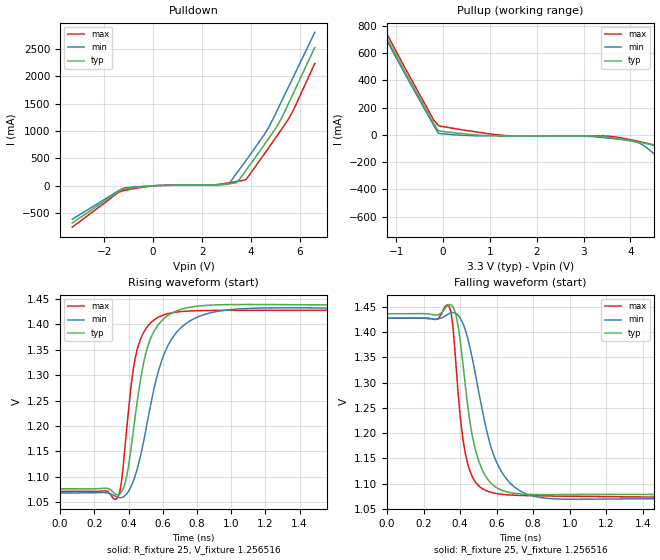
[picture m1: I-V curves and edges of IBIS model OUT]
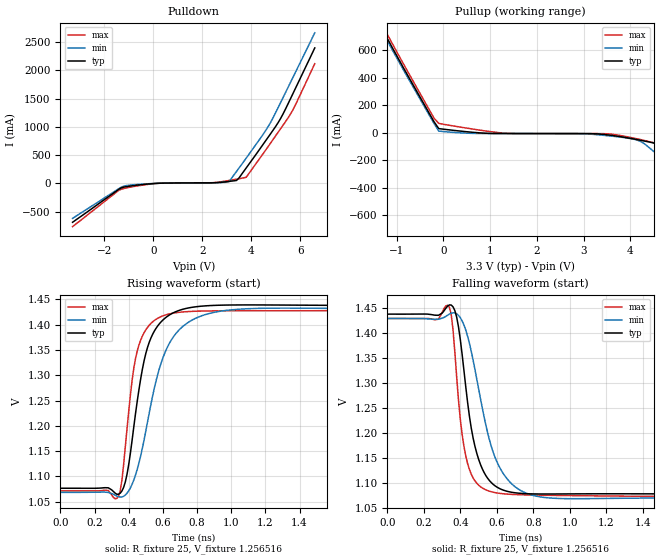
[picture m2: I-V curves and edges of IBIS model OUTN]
|   IBIS File of SG2520VHN C
|   LVDS, Vcc=3.3V, Io=7mA, fo>212.5MHz
[IBIS Ver]   3.2
[File Name]   sg2520vhn_hf_7m_33v.ibs
[File Rev]   1.0
[Date]   July 30, 2020
[Source]
Fairchild Ensigna Lab's Method
[Notes]
Created by Minoru Kozaki
[Disclaimer]
Seiko Epson Corporation makes no warranty with respect to the
information contained herein.
[Copyright]
Copyright(C) 2020, Seiko Epson Corporation. All rights reserved.
|   Component
[Component]   SG2520VHN
[Manufacturer]  Seiko Epson Corporation
[Package]
R_pkg   17.7m   NA   NA
L_pkg   235p   NA   NA
C_pkg   208f   NA   NA
[Pin]   signal_name   model_name   R_pin   L_pin   C_pin
1   OE/ST   NC
2   NC   NC
3   GND   GND
4   OUT   OUT   17.7m   235p   208f
5   OUTN   OUTN   10.4m   129p   221f
6   VCC   POWER
[Diff Pin] inv_pin  vdiff  tdelay_typ
4   5   0   0
| Models and submodels in the file (2): OUT (Output), OUTN (Output)
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|   Model OUT
[Model]   OUT
Model_type   Output
Polarity   Non-Inverting
Vref = 1.25
Vmeas = 1.25
Rref = 25
Cref = 0
C_comp   4.5p   4.5p   4.5p
[Temperature Range]   25   105   -40
[Voltage Range]   3.3   2.97   3.63
[Pullup Reference]   3.3   2.97   3.63
[Pulldown Reference]   0   0   0
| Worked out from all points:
|   slope of the pulldown table from 0 to 0.495 V, typ, clamps not added: 60.1 ohm
|   slope of the pullup table from 0 to 0.495 V, typ, clamps not added: 26.8 ohm
|   falling waveform, R_fixture 25, V_fixture 1.256516: 20-80 % time 92ps typ, 140ps min, 66ps max; typ from 1.44 V to 1.08 V
|   rising waveform, R_fixture 25, V_fixture 1.256516: 20-80 % time 109ps typ, 158ps min, 81.2ps max; typ from 1.08 V to 1.44 V
[Pullup]
-3.3V     2.52A      2.492A     2.553A
-1.4V     837.1mA    817.7mA    870.6mA
-1.3V     772.7mA    753.7mA    805.3mA
-1.2V     708.4mA    690.2mA    740mA
-200mV    81.14mA    68.43mA    107.5mA
-100mV    28.99mA    10.87mA    66.98mA
1.3V      -6.928mA   -7.066mA   -4.25mA
3.7V      -25.31mA   -29.45mA   -16.55mA
4.2V      -55.06mA   -61.12mA   -49.68mA
4.6V      -88.94mA   -164.9mA   -82.59mA
5.1V      -237.8mA   -305.4mA   -156.3mA
6.6V      -698.2mA   -717.4mA   -668.6mA
[Pulldown]
-3.3V     -683.2mA   -614.5mA   -759.8mA
-1.3V     -78.51mA   -64.83mA   -102.6mA
-900mV    -45.62mA   -28.83mA   -63.64mA
100mV     -996uA     -459.2uA   -2.878mA
2.4V      9.207mA    8.749mA    11.16mA
3.1V      34.38mA    33.73mA    50.95mA
3.4V      51.2mA     217.7mA    74.09mA
3.8V      283.8mA    464.4mA    112mA
4.6V      786.4mA    975.9mA    614.4mA
5.2V      1.197A     1.498A     999.8mA
5.7V      1.663A     1.963A     1.357A
6.6V      2.523A     2.802A     2.232A
[Falling Waveform]
R_fixture = 25
V_fixture = 1.256516
V_fixture_min = 1.247959
V_fixture_max = 1.249678
0s        1.437V     1.428V     1.428V
340ps     1.455V     1.437V     1.452V
380ps     1.43V      1.437V     1.323V
410ps     1.355V     1.422V     1.203V
440ps     1.259V     1.39V      1.141V
500ps     1.147V     1.286V     1.096V
580ps     1.097V     1.16V      1.082V
700ps     1.08V      1.092V     1.077V
900ps     1.078V     1.07V      1.075V
4ns       1.077V     1.069V     1.072V
[Rising Waveform]
R_fixture = 25
V_fixture = 1.256516
V_fixture_min = 1.247959
V_fixture_max = 1.249678
0s        1.076V     1.068V     1.071V
320ps     1.067V     1.062V     1.056V
360ps     1.07V      1.059V     1.094V
420ps     1.169V     1.085V     1.293V
450ps     1.246V     1.115V     1.35V
520ps     1.364V     1.226V     1.4V
630ps     1.417V     1.358V     1.421V
780ps     1.435V     1.411V     1.427V
1.05ns    1.439V     1.43V      1.428V
4ns       1.437V     1.428V     1.428V
[Ramp]
R_load = 25
dV/dt_r   0.21562/108.00p   0.21479/156.49p   0.21376/80.76p
dV/dt_f   0.21562/91.62p   0.21479/139.10p   0.21376/65.76p
|   Model OUTN
[Model]   OUTN
Model_type   Output
Polarity   Inverting
Vref = 1.250
Vmeas = 1.250
Rref = 25
Cref = 0
C_comp   4.5p   4.5p   4.5p
[Temperature Range]   25   105   -40
[Voltage Range]   3.3   2.97   3.63
[Pullup Reference]   3.3   2.97   3.63
[Pulldown Reference]   0   0   0
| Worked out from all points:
|   slope of the pulldown table from 0 to 0.495 V, typ, clamps not added: 60 ohm
|   slope of the pullup table from 0 to 0.495 V, typ, clamps not added: 26.9 ohm
|   falling waveform, R_fixture 25, V_fixture 1.256516: 20-80 % time 91.9ps typ, 139ps min, 66.3ps max; typ from 1.44 V to 1.08 V
|   rising waveform, R_fixture 25, V_fixture 1.256516: 20-80 % time 109ps typ, 158ps min, 81.5ps max; typ from 1.08 V to 1.44 V
[Pullup]
-3.3V     2.395A     2.372A     2.423A
-1.4V     808.1mA    789.2mA    840.5mA
-1.3V     745.9mA    727.6mA    777.4mA
-1.2V     683.9mA    666.3mA    714.4mA
-200mV    78.49mA    66.12mA    104.1mA
-100mV    28.93mA    10.86mA    66.77mA
1.3V      -6.928mA   -7.066mA   -4.256mA
3.7V      -25.36mA   -29.54mA   -16.57mA
4.2V      -55.19mA   -61.29mA   -49.83mA
4.6V      -89mA      -165.9mA   -82.88mA
5.1V      -238.9mA   -307.6mA   -155.7mA
6.6V      -703.8mA   -723.9mA   -673.1mA
[Pulldown]
-3.3V     -689.3mA   -620.3mA   -765.7mA
-1.3V     -78.67mA   -65.1mA    -102.7mA
-900mV    -45.7mA    -28.92mA   -63.79mA
100mV     -1.002mA   -463.1uA   -2.889mA
2.4V      9.21mA     8.751mA    11.17mA
3.1V      34.3mA     32.72mA    50.78mA
3.4V      51.07mA    210.2mA    73.82mA
3.8V      274.2mA    448.4mA    108.6mA
4.7V      820.8mA    1.009A     655.1mA
5.2V      1.146A     1.428A     965.6mA
5.7V      1.583A     1.869A     1.297A
6.6V      2.398A     2.666A     2.119A
[Falling Waveform]
R_fixture = 25
V_fixture = 1.256516
V_fixture_min = 1.247959
V_fixture_max = 1.249678
0s        1.437V     1.428V     1.428V
330ps     1.453V     1.435V     1.454V
360ps     1.451V     1.44V      1.406V
400ps     1.386V     1.43V      1.227V
440ps     1.26V      1.393V     1.139V
500ps     1.147V     1.288V     1.096V
580ps     1.097V     1.161V     1.081V
700ps     1.08V      1.092V     1.077V
900ps     1.078V     1.07V      1.075V
4ns       1.077V     1.069V     1.071V
[Rising Waveform]
R_fixture = 25
V_fixture = 1.256516
V_fixture_min = 1.247959
V_fixture_max = 1.249678
0s        1.076V     1.068V     1.071V
320ps     1.067V     1.063V     1.056V
360ps     1.071V     1.059V     1.092V
420ps     1.173V     1.085V     1.291V
450ps     1.25V      1.114V     1.349V
520ps     1.365V     1.226V     1.399V
630ps     1.418V     1.358V     1.421V
780ps     1.435V     1.411V     1.427V
1.05ns    1.439V     1.431V     1.428V
4ns       1.437V     1.428V     1.428V
[Ramp]
R_load = 25
dV/dt_r   0.21531/107.90p   0.21450/155.82p   0.21345/80.94p
dV/dt_f   0.21531/91.30p   0.21450/138.01p   0.21345/65.83p
